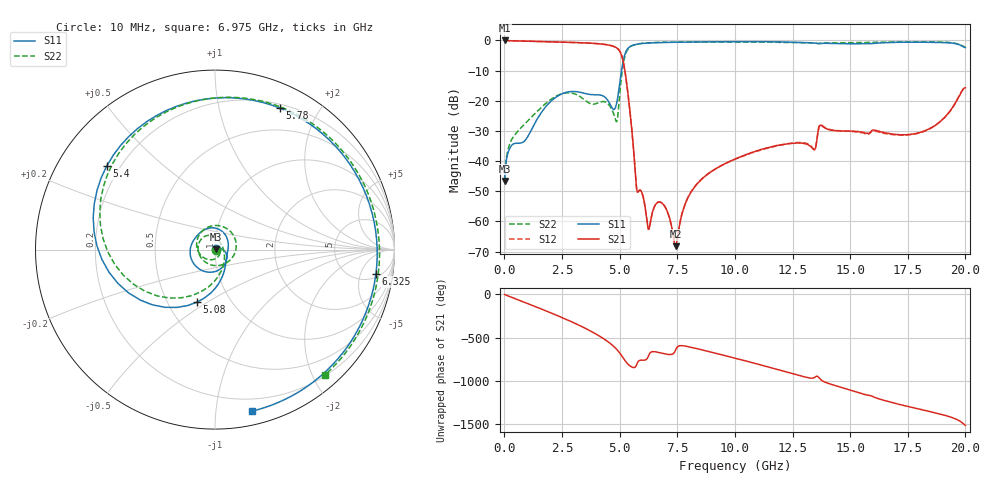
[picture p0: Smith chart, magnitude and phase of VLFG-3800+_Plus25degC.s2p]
! Mini-Circuits
! S2P DATA File Format
! Type: LOW PASS FILTER
! Model: VLFG-3800+
! All S Parameters are in dB deg format
! TEST CONDITIONS: INPUT POWER = 0 dBm @ Temperature = +25 deg C
# MHz S dB R 50
!Frequency  S11 dB  S11 DEG  S21 dB  S21 DEG  S12 dB  S12 DEG  S22 dB  S22 DEG
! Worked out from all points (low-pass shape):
!   900 points, 10 MHz to 20 GHz, reference 50 ohm
!   highest |S21| = -0.04 dB at 10 MHz (marker M1); lowest = -68.2 dB at 7.425 GHz (marker M2)
!   |S21| within 3 dB of the highest: start of sweep to 4.95 GHz
!   lowest |S11| = -46.6 dB at 10 MHz (marker M3), VSWR 1.01, Z = 50.4 + j0.272 ohm
!   |S11| at or under -10 dB: start of sweep to 5.083 GHz
!   |S22| runs from -46.8 to -0.5 dB; largest |S21 - S12| = 0.0057
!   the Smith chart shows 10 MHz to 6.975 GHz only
!   S11 on the Smith chart (normalised r, x): 10 MHz: 1.01, +0.01; 5.08 GHz: 0.70, -0.45; 5.4 GHz: 0.15, +0.33; 5.78 GHz: 0.24, +1.53; 6.325 GHz: 6, -9; 6.975 GHz: 0.10, -1.25
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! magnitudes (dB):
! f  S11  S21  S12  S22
! 10 MHz  -46.6  0.0  0.0  -46.8
! 260 MHz  -35.4  -0.1  -0.1  -33.8
! 1 GHz  -32.1  -0.3  -0.3  -26.8
! 2.12 GHz  -19.5  -0.5  -0.5  -19.0
! 3.35 GHz  -17.3  -0.8  -0.8  -19.0
! 4.42 GHz  -19.3  -1.4  -1.4  -20.6
! 4.84 GHz  -21.8  -2.4  -2.4  -26.7
! 5.08 GHz  -10.2  -4.9  -4.9  -12.1
! 5.4 GHz  -2.4  -20.2  -20.2  -2.5
! 5.78 GHz  -1.2  -50.3  -50.3  -1.2
! 6.325 GHz  -0.9  -60.6  -60.7  -0.8
! 6.675 GHz  -0.8  -53.6  -53.6  -0.7
! 6.975 GHz  -0.7  -55.3  -55.2  -0.6
! 7.425 GHz  -0.6  -68.2  -68.1  -0.6
! 7.8 GHz  -0.6  -55.2  -55.1  -0.6
! 8.225 GHz  -0.5  -48.9  -48.8  -0.6
! 10.03 GHz  -0.4  -39.3  -39.4  -0.6
! 13.35 GHz  -0.8  -35.7  -35.4  -0.9
! 13.85 GHz  -1.0  -28.8  -28.6  -0.9
! 16.68 GHz  -0.7  -30.8  -31.1  -0.6
! 18.62 GHz  -0.7  -28.5  -28.6  -0.5
! 20 GHz  -2.4  -15.7  -15.5  -2.3
